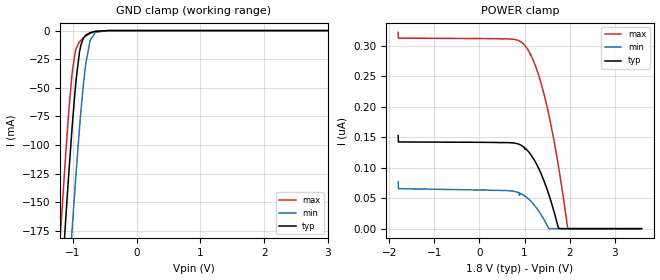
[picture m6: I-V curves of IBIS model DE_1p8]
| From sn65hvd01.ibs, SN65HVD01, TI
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|   Model
[Model]   DE_1p8
Model_type   Input
Vinl = 0.54
Vinh = 1.26
|   typ   min   max
C_comp   0.767pF   0.735pF   0.817pF
[Voltage Range]   1.8   1.62   1.98
[Temperature Range]   27   125   -40
[Power Clamp Reference]   1.8   1.62   1.98
[GND Clamp Reference]   -0   -0   -0
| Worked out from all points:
|   GND clamp passes 1 mA (typ) near -0.67 V on its own axis
[GND Clamp]
|   Voltage   I(typ)   I(min)   I(max)
-1.8V     -806.5mA   -899.9mA   -749.6mA
-1.195V   -236.8mA   -332.4mA   -177.8mA
-1.109V   -161.6mA   -255.8mA   -104.5mA
-1.017V   -87.98mA   -177.7mA   -40.06mA
-963mV    -50.97mA   -134.3mA   -18.55mA
-898.2mV  -19.41mA   -86.34mA   -9.985mA
-871.2mV  -12mA      -68.3mA    -8.312mA
-801mV    -4.122mA   -29.96mA   -5.002mA
-725.4mV  -1.742mA   -7.905mA   -2.41mA
-644.4mV  -602.8uA   -1.467mA   -775.4uA
-450mV    -15.16uA   -36.1uA    -10.16uA
3.595V    0A         0A         0A
[POWER Clamp]
|   Voltage   I(typ)   I(min)   I(max)
-1.8V     152.6nA    77nA       322.1nA
-1.795V   142.2nA    65.61nA    312.6nA
543.6mV   141.3nA    62.62nA    311.6nA
937.8mV   136.2nA    56.73nA    305.7nA
1.067V    128.1nA    50.07nA    294.6nA
1.197V    115nA      40.4nA     275.7nA
1.316V    98.55nA    28.84nA    251.3nA
1.44V     76.75nA    13.88nA    218.5nA
1.543V    55.14nA    0A         185.7nA
1.753V    401.5pA    0A         102.1nA
1.964V    0A         0A         0A
3.595V    0A         0A         0A
